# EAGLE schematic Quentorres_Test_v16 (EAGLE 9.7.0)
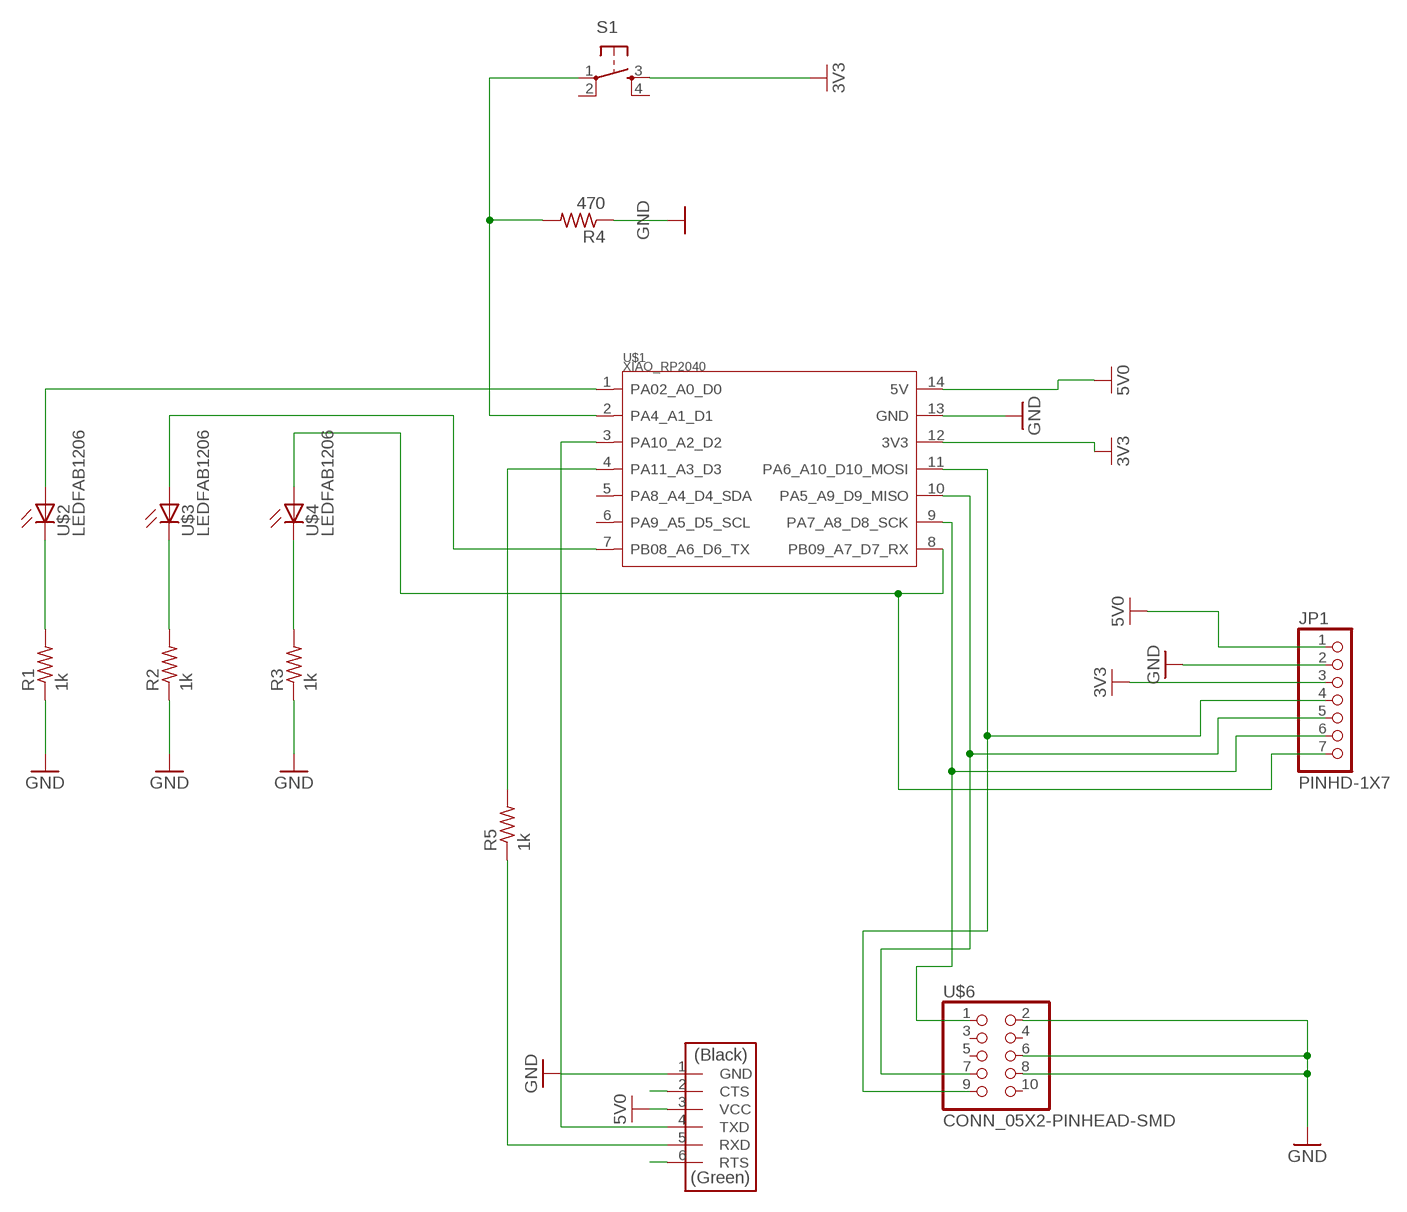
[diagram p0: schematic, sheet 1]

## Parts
JP1  PINHD-1X7  [1X07]
R1  1k  R1206FAB  [R1206FAB]
R2  1k  R1206FAB  [R1206FAB]
R3  1k  R1206FAB  [R1206FAB]
R4  470  R1206FAB  [R1206FAB]
R5  1k  R1206FAB  [R1206FAB]
S1  SW_SWITCH_TACTILE_6MM6MM_SWITCH  [6MM_SWITCH]
U$1  XIAO_RP2040  [XIAO_RP2040_TAPED]
U$2  LEDFAB1206  [LED1206FAB]
U$3  LEDFAB1206  [LED1206FAB]
U$4  LEDFAB1206  [LED1206FAB]
U$5  CONN_06_FTDI-SMD-HEADER  [1X06SMD]
U$6  CONN_05X2-PINHEAD-SMD  [2X05SMD]

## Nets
3V3: JP1.3 S1.3(S) U$1.12(3V3)
5V0: JP1.1 U$1.14(5V) U$5.3(VCC)
GND: JP1.2 R1.1 R2.1 R3.1 R4.1 U$1.13(GND) U$5.1(GND) U$6.2 U$6.6 U$6.8
N$1: R3.2 U$4.2(C)
N$2: R2.2 U$3.2(C)
N$3: R1.2 U$2.2(C)
N$4: U$1.1(PA02_A0_D0) U$2.1(A)
N$5: U$1.7(PB08_A6_D6_TX) U$3.1(A)
N$6: JP1.7 U$1.8(PB09_A7_D7_RX) U$4.1(A)
N$7: R4.2 S1.1(P) U$1.2(PA4_A1_D1)
N$8: JP1.4 U$1.11(PA6_A10_D10_MOSI) U$6.9
N$9: JP1.5 U$1.10(PA5_A9_D9_MISO) U$6.7
N$10: JP1.6 U$1.9(PA7_A8_D8_SCK) U$6.1
N$11: U$5.2(CTS)
N$12: U$1.3(PA10_A2_D2) U$5.4(TXD)
N$13: R5.2 U$1.4(PA11_A3_D3)
N$14: R5.1 U$5.5(RXD)
N$16: U$5.6(RTS)
Unconnected: S1.2(P1) S1.4(S1) U$1.5(PA8_A4_D4_SDA) U$1.6(PA9_A5_D5_SCL) U$6.3 U$6.4 U$6.5 U$6.10

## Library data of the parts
JP1 = Connector:PINHD-1X7: PIN HEADER; CATEGORY: Headers; DESCRIPTION: Header-Straight-7 Position; PACKAGE_TYPE: THT; PITCH: 0.100" (2.54mm); SUBCATEGORY: Headers-Male Pins; TYPE: Board to Board or Cable-Unshrouded-Through Hole-Straight
R1-R5 = fab:R: Resistor (US Symbol)
S1 = fab:SW_SWITCH_TACTILE_6MM: OMRON SWITCH
U$1 = fab:XIAO_RP2040
U$2-U$4 = fab:LED: LED
U$5 = fab:CONN_06_FTDI-SMD-HEADER
U$6 = fab:CONN_05X2-PINHEAD-SMD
